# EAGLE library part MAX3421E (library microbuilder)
MAX3421E SPI-Interface USB Device/Host Controller Digikey: MAX3421EETJ+-ND
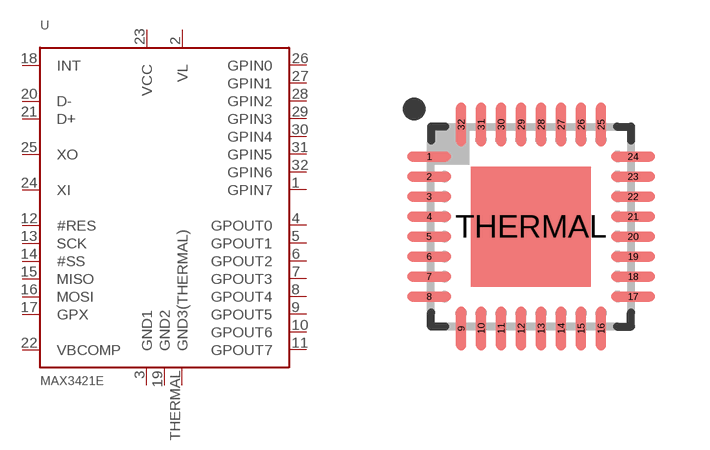
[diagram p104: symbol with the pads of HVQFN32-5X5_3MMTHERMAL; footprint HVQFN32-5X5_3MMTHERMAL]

Designator prefix U

## MAX3421E  [HVQFN32-5X5_3MMTHERMAL]
1  GPIN7  in
2  VL  pwr
3  GND1  pwr
4  GPOUT0  out
5  GPOUT1  out
6  GPOUT2  out
7  GPOUT3  out
8  GPOUT4  out
9  GPOUT5  out
10  GPOUT6  out
11  GPOUT7  out
12  #RES
13  SCK
14  #SS
15  MISO
16  MOSI
17  GPX
18  INT
19  GND2  pwr
20  D-
21  D+
22  VBCOMP
23  VCC  pwr
24  XI
25  XO
26  GPIN0  in
27  GPIN1  in
28  GPIN2  in
29  GPIN3  in
30  GPIN4  in
31  GPIN5  in
32  GPIN6  in
THERMAL  GND3(THERMAL)  pwr

## Footprint HVQFN32-5X5_3MMTHERMAL (pad centres in mm)
smd 1.1 x 0.25: 1 -2.55,1.75; 2 -2.55,1.25; 3 -2.55,0.75; 4 -2.55,0.25; 5 -2.55,-0.25; 6 -2.55,-0.75; 7 -2.55,-1.25; 8 -2.55,-1.75; 17 2.55,-1.75; 18 2.55,-1.25; 19 2.55,-0.75; 20 2.55,-0.25; 21 2.55,0.25; 22 2.55,0.75; 23 2.55,1.25; 24 2.55,1.75
smd 0.25 x 1.1: 9 -1.75,-2.55; 10 -1.25,-2.55; 11 -0.75,-2.55; 12 -0.25,-2.55; 13 0.25,-2.55; 14 0.75,-2.55; 15 1.25,-2.55; 16 1.75,-2.55; 25 1.75,2.55; 26 1.25,2.55; 27 0.75,2.55; 28 0.25,2.55; 29 -0.25,2.55; 30 -0.75,2.55; 31 -1.25,2.55; 32 -1.75,2.55
smd 3 x 3: THERMAL 0,0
